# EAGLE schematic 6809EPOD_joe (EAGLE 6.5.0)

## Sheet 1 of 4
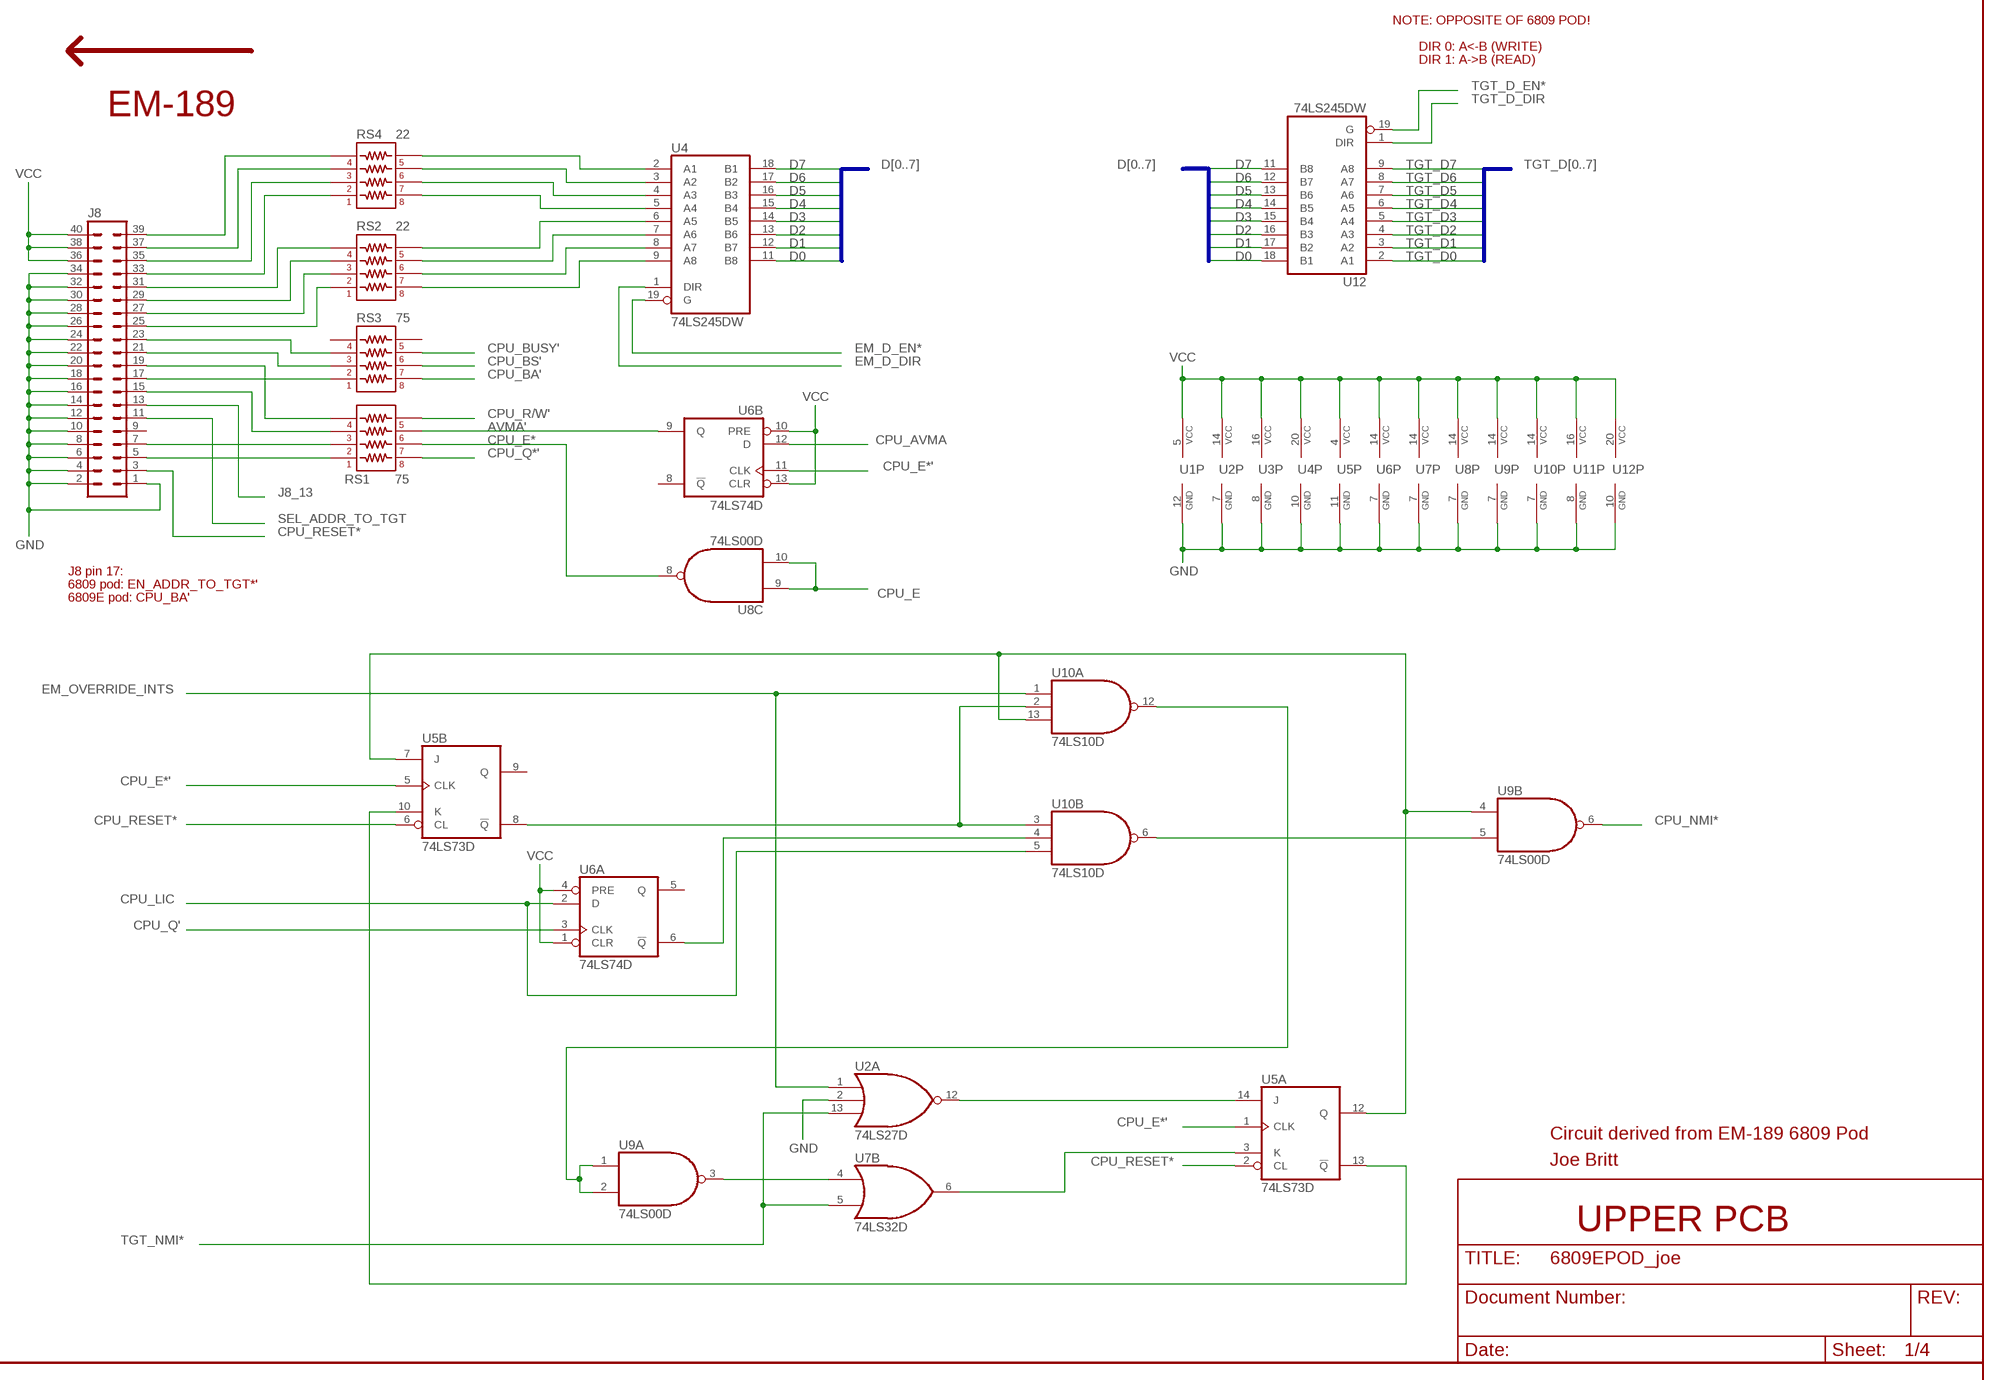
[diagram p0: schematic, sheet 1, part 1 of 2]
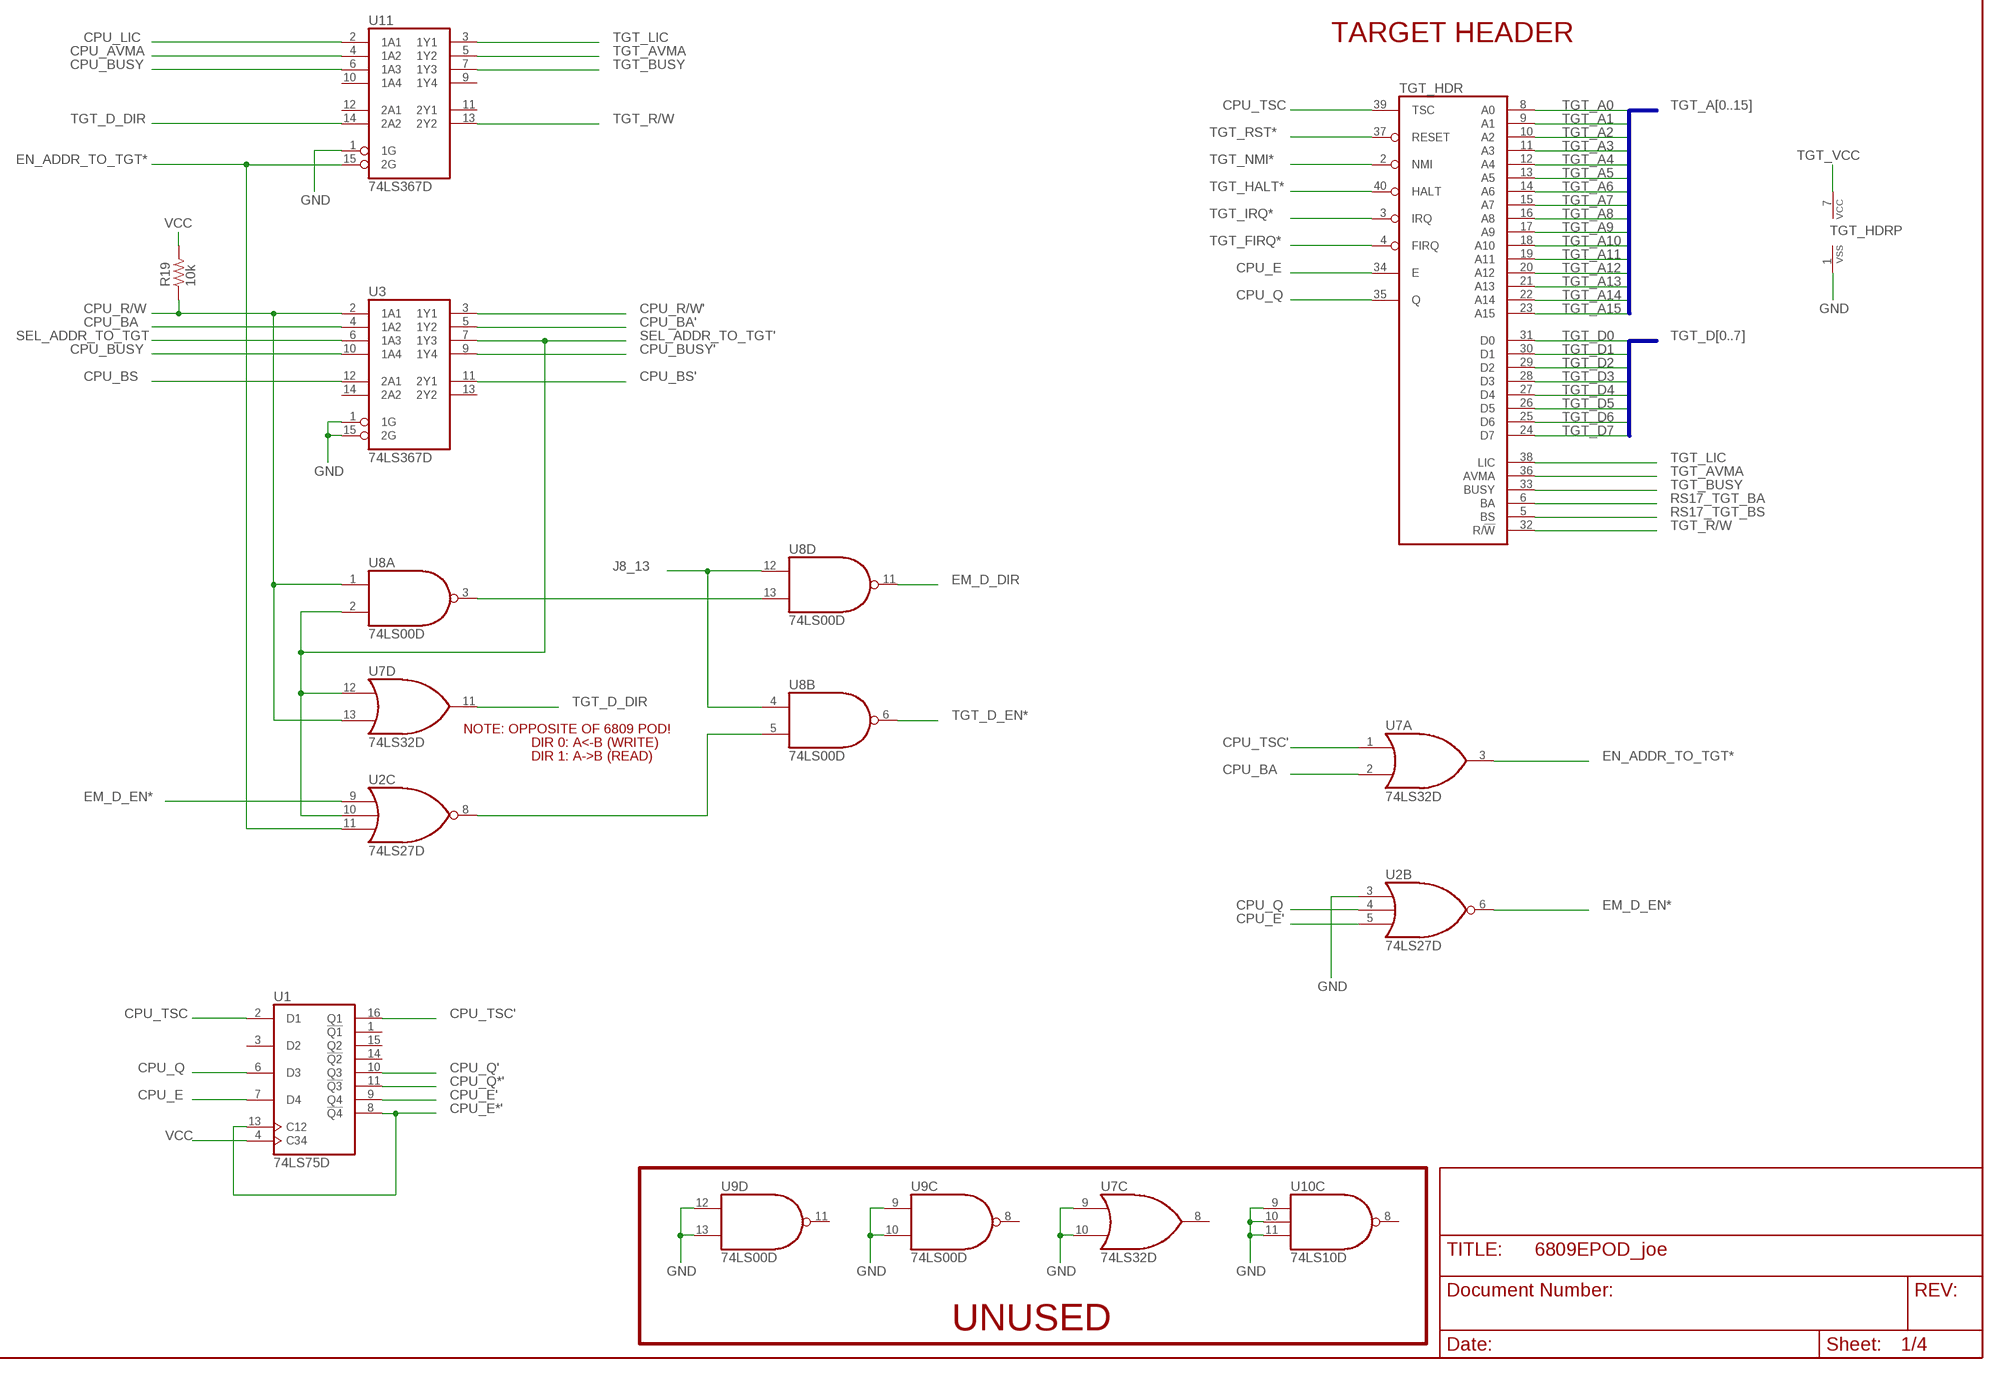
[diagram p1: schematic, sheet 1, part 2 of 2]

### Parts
J8  MA20-2  [MA20-2]
R19  10k  R_0603  [R0603]
RS1  75  V8V  [V8V]
RS2  22  V8V  [V8V]
RS3  75  V8V  [V8V]
RS4  22  V8V  [V8V]
TGT_HDR  6809EHDR40  [HDR40]
U1  74LS75D  [SO16]
U2  74LS27D  [SO14]
U3  74LS367D  [SO16]
U4  74LS245DW  [SO20W]
U5  74LS73D  [SO14]
U6  74LS74D  [SO14]
U7  74LS32D  [SO14]
U8  74LS00D  [SO14]
U9  74LS00D  [SO14]
U10  74LS10D  [SO14]
U11  74LS367D  [SO16]
U12  74LS245DW  [SO20W]

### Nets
AVMA': RS1.R3B U6.9(B:Q)
CPU_AVMA: U6.12(B:D) U11.4(1A2) ; also sheet 2
CPU_BA: U3.4(1A2) U7.2(A:I1) ; also sheet 2
CPU_BA': RS3.R1B U3.5(1Y2)
CPU_BS: U3.12(2A1) ; also sheet 2
CPU_BS': RS3.R2B U3.11(2Y1)
CPU_BUSY: U3.10(1A4) U11.6(1A3) ; also sheet 2
CPU_BUSY': RS3.R3B U3.9(1Y4)
CPU_E: TGT_HDR.34(E) U1.7(D4) U8.9(C:I0) U8.10(C:I1) ; also sheet 2
CPU_E': U1.9(Q4) U2.5(B:I2)
CPU_E*: RS1.R2B U8.8(C:O)
CPU_E*': U1.8(!Q4) U1.13(C12) U5.1(A:CLK) U5.5(B:CLK) U6.11(B:CLK)
CPU_LIC: U6.2(A:D) U10.5(B:I2) U11.2(1A1) ; also sheet 2
CPU_NMI*: U9.6(B:O) ; also sheet 2
CPU_Q: TGT_HDR.35(Q) U1.6(D3) U2.4(B:I1) ; also sheet 2
CPU_Q': U1.10(Q3) U6.3(A:CLK)
CPU_Q*': RS1.R1B U1.11(!Q3)
CPU_R/W: R19.1 U3.2(1A1) U7.13(D:I1) U8.1(A:I0) ; also sheet 2
CPU_R/W': RS1.R4B U3.3(1Y1)
CPU_RESET*: J8.3 U5.2(A:CL) U5.6(B:CL) ; also sheet 2
CPU_TSC: TGT_HDR.39(TSC) U1.2(D1) ; also sheet 2
CPU_TSC': U1.16(Q1) U7.1(A:I0)
D0: U4.11(B8) U12.18(B1) ; also sheet 2
D1: U4.12(B7) U12.17(B2) ; also sheet 2
D2: U4.13(B6) U12.16(B3) ; also sheet 2
D3: U4.14(B5) U12.15(B4) ; also sheet 2
D4: U4.15(B4) U12.14(B5) ; also sheet 2
D5: U4.16(B3) U12.13(B6) ; also sheet 2
D6: U4.17(B2) U12.12(B7) ; also sheet 2
D7: U4.18(B1) U12.11(B8) ; also sheet 2
EM_D_DIR: U4.1(DIR) U8.11(D:O)
EM_D_EN*: U2.6(B:O) U2.9(C:I0) U4.19(G)
EM_OVERRIDE_INTS: U2.1(A:I0) U10.1(A:I0) ; also sheet 2
EN_ADDR_TO_TGT*: U2.11(C:I2) U7.3(A:O) U11.15(2G) ; also sheet 2
GND: J8.1 J8.2 J8.4 J8.6 J8.8 J8.10 J8.12 J8.14 J8.16 J8.18 J8.20 J8.22 J8.24 J8.26 J8.28 J8.30 J8.32 J8.34 TGT_HDR.1(VSS) U1.12(GND) U2.2(A:I1) U2.3(B:I0) U2.7(P:GND) U3.1(1G) U3.8(GND) U3.15(2G) U4.10(GND) U5.11(P:GND) U6.7(P:GND) U7.7(P:GND) U7.9(C:I0) U7.10(C:I1) U8.7(P:GND) U9.7(P:GND) U9.9(C:I0) U9.10(C:I1) U9.12(D:I0) U9.13(D:I1) U10.7(P:GND) U10.9(C:I0) U10.10(C:I1) U10.11(C:I2) U11.1(1G) U11.8(GND) U12.10(GND) ; also sheet 2,3
J8_13: J8.13 U8.4(B:I0) U8.12(D:I0)
N$2: J8.5 RS1.R1A
N$3: J8.7 RS1.R2A
N$4: J8.15 RS1.R3A
N$5: J8.19 RS1.R4A
N$6: J8.17 RS3.R1A
N$7: J8.21 RS3.R2A
N$8: J8.23 RS3.R3A
N$9: J8.25 RS2.R1A
N$10: J8.27 RS2.R2A
N$11: J8.29 RS2.R3A
N$12: J8.31 RS2.R4A
N$13: J8.33 RS4.R1A
N$14: J8.35 RS4.R2A
N$15: J8.37 RS4.R3A
N$16: J8.39 RS4.R4A
N$17: RS2.R1B U4.9(A8)
N$18: RS2.R2B U4.8(A7)
N$19: RS2.R3B U4.7(A6)
N$20: RS2.R4B U4.6(A5)
N$21: RS4.R1B U4.5(A4)
N$22: RS4.R2B U4.4(A3)
N$23: RS4.R3B U4.3(A2)
N$24: RS4.R4B U4.2(A1)
N$45: U8.3(A:O) U8.13(D:I1)
N$46: U2.8(C:O) U8.5(B:I1)
N$124: U2.12(A:O) U5.14(A:J)
N$125: U5.8(B:!Q) U10.2(A:I1) U10.3(B:I0)
N$126: U6.6(A:!Q) U10.4(B:I1)
N$127: U5.10(B:K) U5.13(A:!Q)
N$128: U9.5(B:I1) U10.6(B:O)
N$129: U5.7(B:J) U5.12(A:Q) U9.4(B:I0) U10.13(A:I2)
N$130: U9.1(A:I0) U9.2(A:I1) U10.12(A:O)
N$131: U7.4(B:I0) U9.3(A:O)
N$132: U5.3(A:K) U7.6(B:O)
RS17_TGT_BA: TGT_HDR.6(BA) ; also sheet 2
RS17_TGT_BS: TGT_HDR.5(BS) ; also sheet 2
SEL_ADDR_TO_TGT: J8.11 U3.6(1A3)
SEL_ADDR_TO_TGT': U2.10(C:I1) U3.7(1Y3) U7.12(D:I0) U8.2(A:I1) ; also sheet 2
TGT_A0: TGT_HDR.8(A0) ; also sheet 2
TGT_A1: TGT_HDR.9(A1) ; also sheet 2
TGT_A2: TGT_HDR.10(A2) ; also sheet 2
TGT_A3: TGT_HDR.11(A3) ; also sheet 2
TGT_A4: TGT_HDR.12(A4) ; also sheet 2
TGT_A5: TGT_HDR.13(A5) ; also sheet 2
TGT_A6: TGT_HDR.14(A6) ; also sheet 2
TGT_A7: TGT_HDR.15(A7) ; also sheet 2
TGT_A8: TGT_HDR.16(A8) ; also sheet 2
TGT_A9: TGT_HDR.17(A9) ; also sheet 2
TGT_A10: TGT_HDR.18(A10) ; also sheet 2
TGT_A11: TGT_HDR.19(A11) ; also sheet 2
TGT_A12: TGT_HDR.20(A12) ; also sheet 2
TGT_A13: TGT_HDR.21(A13) ; also sheet 2
TGT_A14: TGT_HDR.22(A14) ; also sheet 2
TGT_A15: TGT_HDR.23(A15) ; also sheet 2
TGT_AVMA: TGT_HDR.36(AVMA) U11.5(1Y2)
TGT_BUSY: TGT_HDR.33(BUSY) U11.7(1Y3)
TGT_D0: TGT_HDR.31(D0) U12.2(A1)
TGT_D1: TGT_HDR.30(D1) U12.3(A2)
TGT_D2: TGT_HDR.29(D2) U12.4(A3)
TGT_D3: TGT_HDR.28(D3) U12.5(A4)
TGT_D4: TGT_HDR.27(D4) U12.6(A5)
TGT_D5: TGT_HDR.26(D5) U12.7(A6)
TGT_D6: TGT_HDR.25(D6) U12.8(A7)
TGT_D7: TGT_HDR.24(D7) U12.9(A8)
TGT_D_DIR: U7.11(D:O) U11.14(2A2) U12.1(DIR)
TGT_D_EN*: U8.6(B:O) U12.19(G)
TGT_FIRQ*: TGT_HDR.4(FIRQ) ; also sheet 2
TGT_HALT*: TGT_HDR.40(HALT) ; also sheet 2
TGT_IRQ*: TGT_HDR.3(IRQ) ; also sheet 2
TGT_LIC: TGT_HDR.38(LIC) U11.3(1Y1)
TGT_NMI*: TGT_HDR.2(NMI) U2.13(A:I2) U7.5(B:I1) ; also sheet 2
TGT_R/W: TGT_HDR.32(R/!W) U11.13(2Y2)
TGT_RST*: TGT_HDR.37(RESET) ; also sheet 2
TGT_VCC: TGT_HDR.7(VCC) ; also sheet 2,3
VCC: J8.36 J8.38 J8.40 R19.2 U1.4(C34) U1.5(VCC) U2.14(P:VCC) U3.16(VCC) U4.20(VCC) U5.4(P:VCC) U6.1(A:CLR) U6.4(A:PRE) U6.10(B:PRE) U6.13(B:CLR) U6.14(P:VCC) U7.14(P:VCC) U8.14(P:VCC) U9.14(P:VCC) U10.14(P:VCC) U11.16(VCC) U12.20(VCC) ; also sheet 2,3
Unconnected: J8.9 RS3.R4A RS3.R4B U1.1(!Q1) U1.3(D2) U1.14(!Q2) U1.15(Q2) U3.13(2Y2) U3.14(2A2) U5.9(B:Q) U6.5(A:Q) U6.8(B:!Q) U7.8(C:O) U9.8(C:O) U9.11(D:O) U10.8(C:O) U11.9(1Y4) U11.10(1A4) U11.11(2Y1) U11.12(2A1)

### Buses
D[0..7]
TGT_D[0..7]
TGT_A[0..15]

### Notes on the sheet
- NOTE: OPPOSITE OF 6809 POD!
- DIR 0: A<-B (WRITE)
- DIR 1: A->B (READ)
- EM-189
- J8 pin 17:
- 6809 pod: EN_ADDR_TO_TGT*'
- 6809E pod: CPU_BA'
- Circuit derived from EM-189 6809 Pod
- Joe Britt
- UPPER PCB
- TARGET HEADER
- NOTE: OPPOSITE OF 6809 POD!
- DIR 0: A<-B (WRITE)
- DIR 1: A->B (READ)
- UNUSED

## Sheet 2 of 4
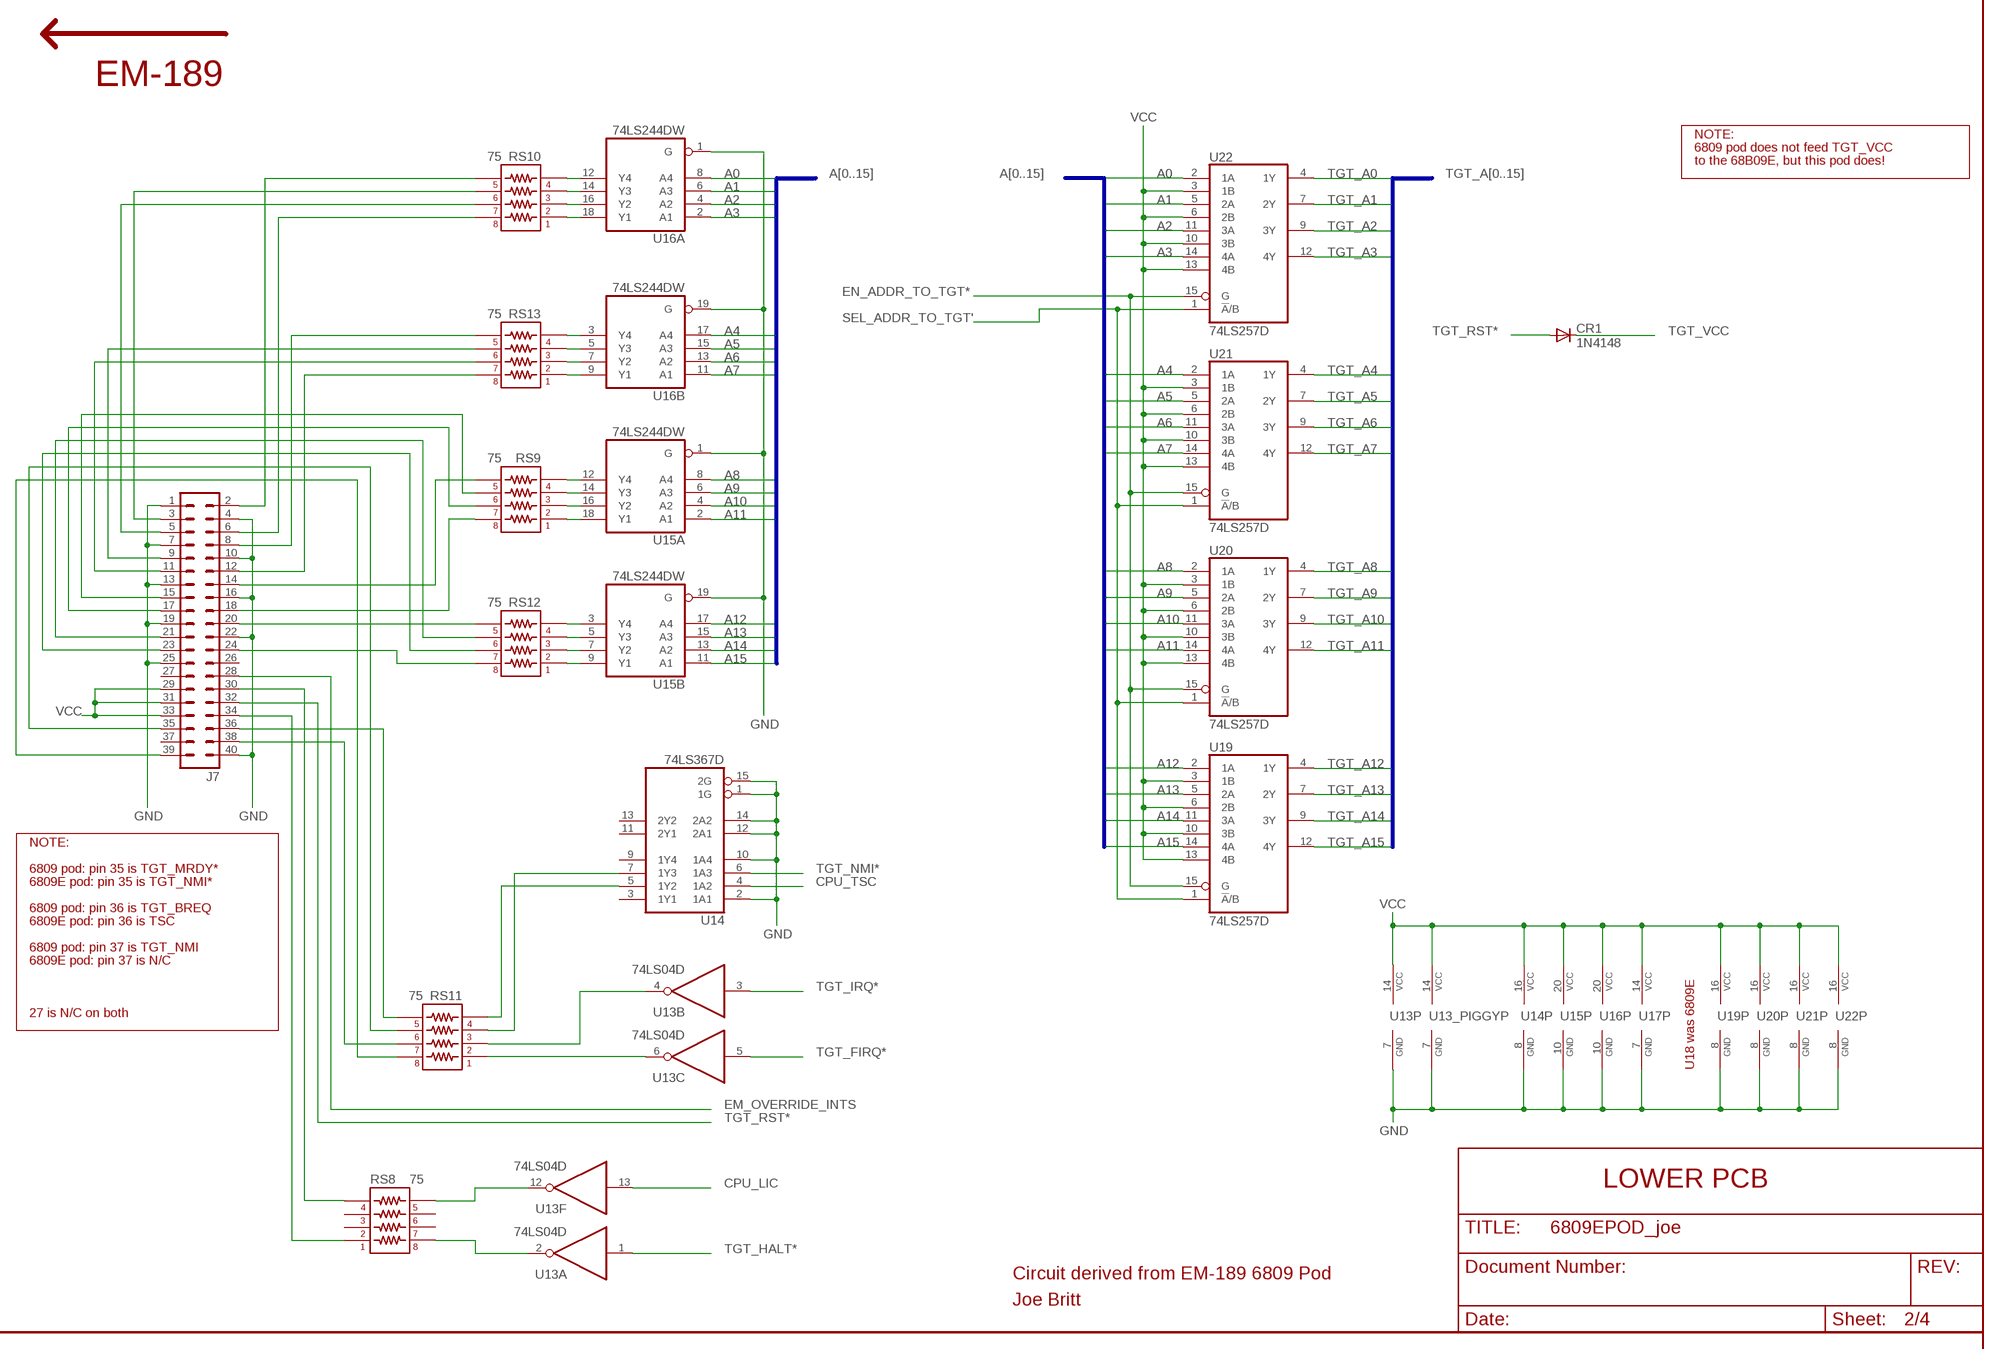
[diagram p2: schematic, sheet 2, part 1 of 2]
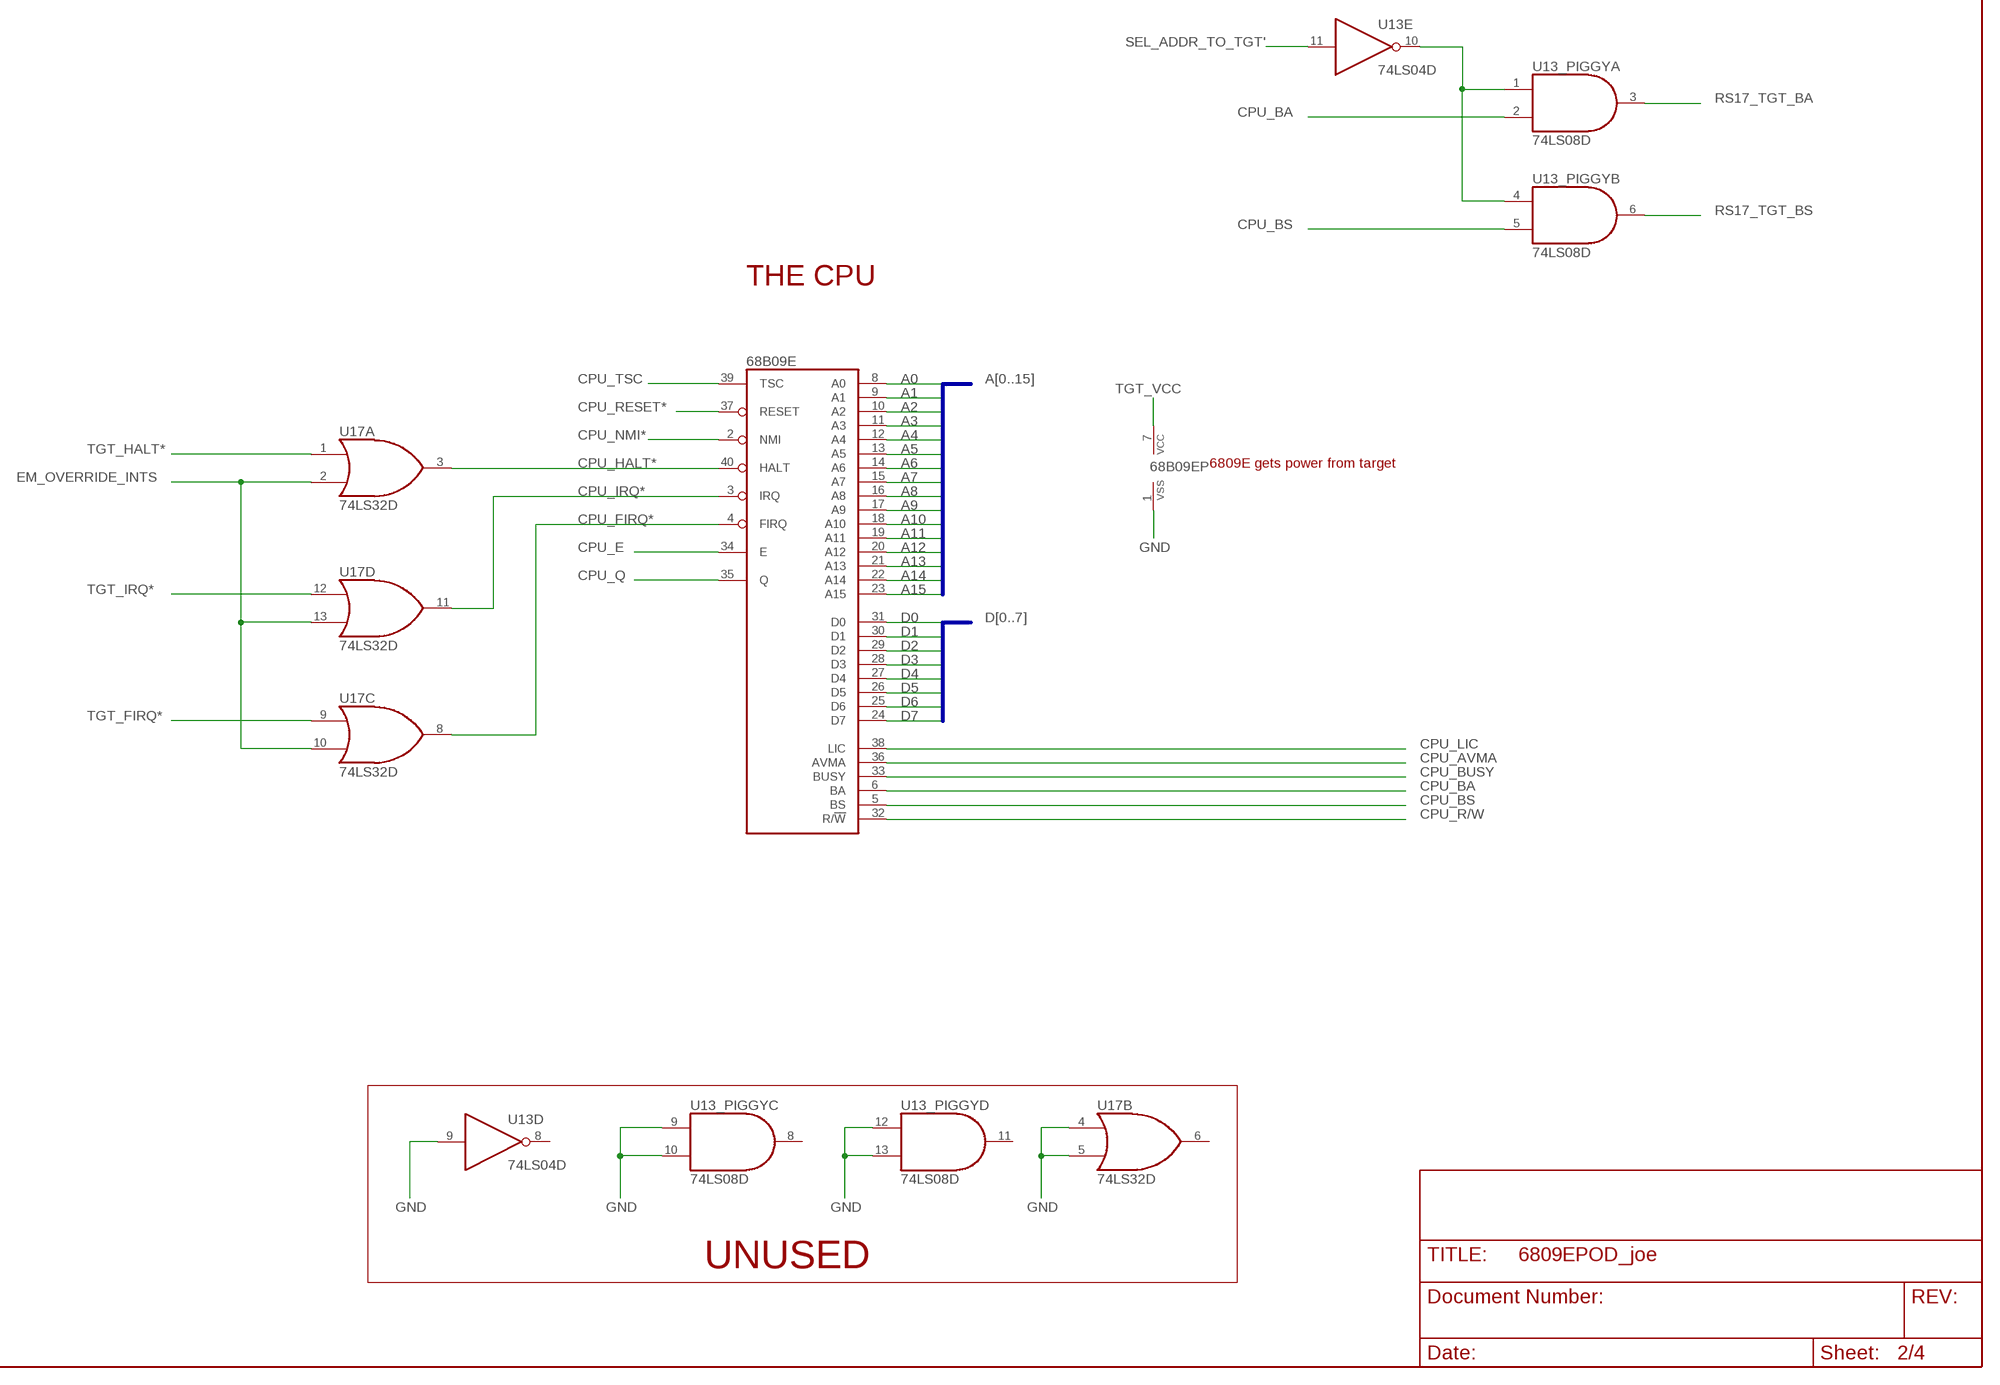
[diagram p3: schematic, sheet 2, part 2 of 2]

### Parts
68B09E  6809EDIP40  [DIL40]
CR1  1N4148  [DO35-10]
J7  MA20-2  [MA20-2]
RS8  75  V8V  [V8V]
RS9  75  V8V  [V8V]
RS10  75  V8V  [V8V]
RS11  75  V8V  [V8V]
RS12  75  V8V  [V8V]
RS13  75  V8V  [V8V]
U13  74LS04D  [SO14]
U13_PIGGY  74LS08D  [SO14]
U14  74LS367D  [SO16]
U15  74LS244DW  [SO20W]
U16  74LS244DW  [SO20W]
U17  74LS32D  [SO14]
U19  74LS257D  [SO16]
U20  74LS257D  [SO16]
U21  74LS257D  [SO16]
U22  74LS257D  [SO16]

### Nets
A0: 68B09E.8(A0) U16.8(A:A4) U22.2(1A)
A1: 68B09E.9(A1) U16.6(A:A3) U22.5(2A)
A2: 68B09E.10(A2) U16.4(A:A2) U22.11(3A)
A3: 68B09E.11(A3) U16.2(A:A1) U22.14(4A)
A4: 68B09E.12(A4) U16.17(B:A4) U21.2(1A)
A5: 68B09E.13(A5) U16.15(B:A3) U21.5(2A)
A6: 68B09E.14(A6) U16.13(B:A2) U21.11(3A)
A7: 68B09E.15(A7) U16.11(B:A1) U21.14(4A)
A8: 68B09E.16(A8) U15.8(A:A4) U20.2(1A)
A9: 68B09E.17(A9) U15.6(A:A3) U20.5(2A)
A10: 68B09E.18(A10) U15.4(A:A2) U20.11(3A)
A11: 68B09E.19(A11) U15.2(A:A1) U20.14(4A)
A12: 68B09E.20(A12) U15.17(B:A4) U19.2(1A)
A13: 68B09E.21(A13) U15.15(B:A3) U19.5(2A)
A14: 68B09E.22(A14) U15.13(B:A2) U19.11(3A)
A15: 68B09E.23(A15) U15.11(B:A1) U19.14(4A)
CPU_AVMA: 68B09E.36(AVMA) ; also sheet 1
CPU_BA: 68B09E.6(BA) U13_PIGGY.2(A:I1) ; also sheet 1
CPU_BS: 68B09E.5(BS) U13_PIGGY.5(B:I1) ; also sheet 1
CPU_BUSY: 68B09E.33(BUSY) ; also sheet 1
CPU_E: 68B09E.34(E) ; also sheet 1
CPU_FIRQ*: 68B09E.4(FIRQ) U17.8(C:O)
CPU_HALT*: 68B09E.40(HALT) U17.3(A:O)
CPU_IRQ*: 68B09E.3(IRQ) U17.11(D:O)
CPU_LIC: 68B09E.38(LIC) U13.13(F:I) ; also sheet 1
CPU_NMI*: 68B09E.2(NMI) ; also sheet 1
CPU_Q: 68B09E.35(Q) ; also sheet 1
CPU_R/W: 68B09E.32(R/!W) ; also sheet 1
CPU_RESET*: 68B09E.37(RESET) ; also sheet 1
CPU_TSC: 68B09E.39(TSC) U14.4(1A2) ; also sheet 1
D0: 68B09E.31(D0) ; also sheet 1
D1: 68B09E.30(D1) ; also sheet 1
D2: 68B09E.29(D2) ; also sheet 1
D3: 68B09E.28(D3) ; also sheet 1
D4: 68B09E.27(D4) ; also sheet 1
D5: 68B09E.26(D5) ; also sheet 1
D6: 68B09E.25(D6) ; also sheet 1
D7: 68B09E.24(D7) ; also sheet 1
EM_OVERRIDE_INTS: J7.28 U17.2(A:I1) U17.10(C:I1) U17.13(D:I1) ; also sheet 1
EN_ADDR_TO_TGT*: U19.15(G) U20.15(G) U21.15(G) U22.15(G) ; also sheet 1
GND: 68B09E.1(VSS) J7.1 J7.4 J7.7 J7.10 J7.13 J7.16 J7.19 J7.22 J7.25 J7.40 U13.7(P:GND) U13.9(D:I) U13_PIGGY.7(P:GND) U13_PIGGY.9(C:I0) U13_PIGGY.10(C:I1) U13_PIGGY.12(D:I0) U13_PIGGY.13(D:I1) U14.1(1G) U14.2(1A1) U14.8(GND) U14.10(1A4) U14.12(2A1) U14.14(2A2) U14.15(2G) U15.1(A:G) U15.10(P:GND) U15.19(B:G) U16.1(A:G) U16.10(P:GND) U16.19(B:G) U17.4(B:I0) U17.5(B:I1) U17.7(P:GND) U19.8(GND) U20.8(GND) U21.8(GND) U22.8(GND) ; also sheet 1,3
N$61: J7.3 RS10.R3B
N$62: J7.5 RS10.R2B
N$81: J7.9 RS13.R3B
N$82: J7.11 RS13.R2B
N$83: J7.15 RS9.R3B
N$84: J7.17 RS9.R2B
N$85: J7.21 RS12.R3B
N$86: J7.23 RS12.R2B
N$87: J7.35 RS11.R3B
N$88: J7.39 RS11.R1B
N$89: J7.2 RS10.R4B
N$90: J7.6 RS10.R1B
N$91: J7.8 RS13.R4B
N$92: J7.12 RS13.R1B
N$93: J7.18 RS9.R1B
N$94: J7.14 RS9.R4B
N$95: J7.20 RS12.R4B
N$96: J7.24 RS12.R1B
N$97: J7.30 RS8.R4A
N$98: J7.34 RS8.R1A
N$99: J7.36 RS11.R4B
N$100: J7.38 RS11.R2B
N$101: RS10.R4A U16.12(A:Y4)
N$102: RS10.R3A U16.14(A:Y3)
N$103: RS10.R2A U16.16(A:Y2)
N$104: RS10.R1A U16.18(A:Y1)
N$105: RS13.R4A U16.3(B:Y4)
N$106: RS13.R3A U16.5(B:Y3)
N$107: RS13.R2A U16.7(B:Y2)
N$108: RS13.R1A U16.9(B:Y1)
N$109: RS9.R4A U15.12(A:Y4)
N$110: RS9.R3A U15.14(A:Y3)
N$111: RS9.R2A U15.16(A:Y2)
N$112: RS9.R1A U15.18(A:Y1)
N$113: RS12.R4A U15.3(B:Y4)
N$114: RS12.R3A U15.5(B:Y3)
N$115: RS12.R2A U15.7(B:Y2)
N$116: RS12.R1A U15.9(B:Y1)
N$117: U13.10(E:O) U13_PIGGY.1(A:I0) U13_PIGGY.4(B:I0)
N$118: RS8.R1B U13.2(A:O)
N$119: RS11.R2A U13.4(B:O)
N$120: RS11.R1A U13.6(C:O)
N$121: RS8.R4B U13.12(F:O)
N$122: RS11.R4A U14.5(1Y2)
N$123: RS11.R3A U14.7(1Y3)
RS17_TGT_BA: U13_PIGGY.3(A:O) ; also sheet 1
RS17_TGT_BS: U13_PIGGY.6(B:O) ; also sheet 1
SEL_ADDR_TO_TGT': U13.11(E:I) U19.1(!A!/B) U20.1(!A!/B) U21.1(!A!/B) U22.1(!A!/B) ; also sheet 1
TGT_A0: U22.4(1Y) ; also sheet 1
TGT_A1: U22.7(2Y) ; also sheet 1
TGT_A2: U22.9(3Y) ; also sheet 1
TGT_A3: U22.12(4Y) ; also sheet 1
TGT_A4: U21.4(1Y) ; also sheet 1
TGT_A5: U21.7(2Y) ; also sheet 1
TGT_A6: U21.9(3Y) ; also sheet 1
TGT_A7: U21.12(4Y) ; also sheet 1
TGT_A8: U20.4(1Y) ; also sheet 1
TGT_A9: U20.7(2Y) ; also sheet 1
TGT_A10: U20.9(3Y) ; also sheet 1
TGT_A11: U20.12(4Y) ; also sheet 1
TGT_A12: U19.4(1Y) ; also sheet 1
TGT_A13: U19.7(2Y) ; also sheet 1
TGT_A14: U19.9(3Y) ; also sheet 1
TGT_A15: U19.12(4Y) ; also sheet 1
TGT_FIRQ*: U13.5(C:I) U17.9(C:I0) ; also sheet 1
TGT_HALT*: U13.1(A:I) U17.1(A:I0) ; also sheet 1
TGT_IRQ*: U13.3(B:I) U17.12(D:I0) ; also sheet 1
TGT_NMI*: U14.6(1A3) ; also sheet 1
TGT_RST*: CR1.A J7.32 ; also sheet 1
TGT_VCC: 68B09E.7(VCC) CR1.C ; also sheet 1,3
VCC: J7.29 J7.31 J7.33 U13.14(P:VCC) U13_PIGGY.14(P:VCC) U14.16(VCC) U15.20(P:VCC) U16.20(P:VCC) U17.14(P:VCC) U19.3(1B) U19.6(2B) U19.10(3B) U19.13(4B) U19.16(VCC) U20.3(1B) U20.6(2B) U20.10(3B) U20.13(4B) U20.16(VCC) U21.3(1B) U21.6(2B) U21.10(3B) U21.13(4B) U21.16(VCC) U22.3(1B) U22.6(2B) U22.10(3B) U22.13(4B) U22.16(VCC) ; also sheet 1,3
Unconnected: J7.26 J7.27 J7.37 RS8.R2A RS8.R2B RS8.R3A RS8.R3B U13.8(D:O) U13_PIGGY.8(C:O) U13_PIGGY.11(D:O) U14.3(1Y1) U14.9(1Y4) U14.11(2Y1) U14.13(2Y2) U17.6(B:O)

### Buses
A[0..15]
D[0..7]
TGT_A[0..15]

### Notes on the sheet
- EM-189
- NOTE:
- 6809 pod does not feed TGT_VCC
- to the 68B09E, but this pod does!
- NOTE:
- 6809 pod: pin 35 is TGT_MRDY*
- 6809E pod: pin 35 is TGT_NMI*
- 6809 pod: pin 36 is TGT_BREQ
- 6809E pod: pin 36 is TSC
- 6809 pod: pin 37 is TGT_NMI
- 6809E pod: pin 37 is N/C
- 27 is N/C on both
- U18 was 6809E
- LOWER PCB
- Circuit derived from EM-189 6809 Pod
- Joe Britt
- THE CPU
- 6809E gets power from target
- UNUSED

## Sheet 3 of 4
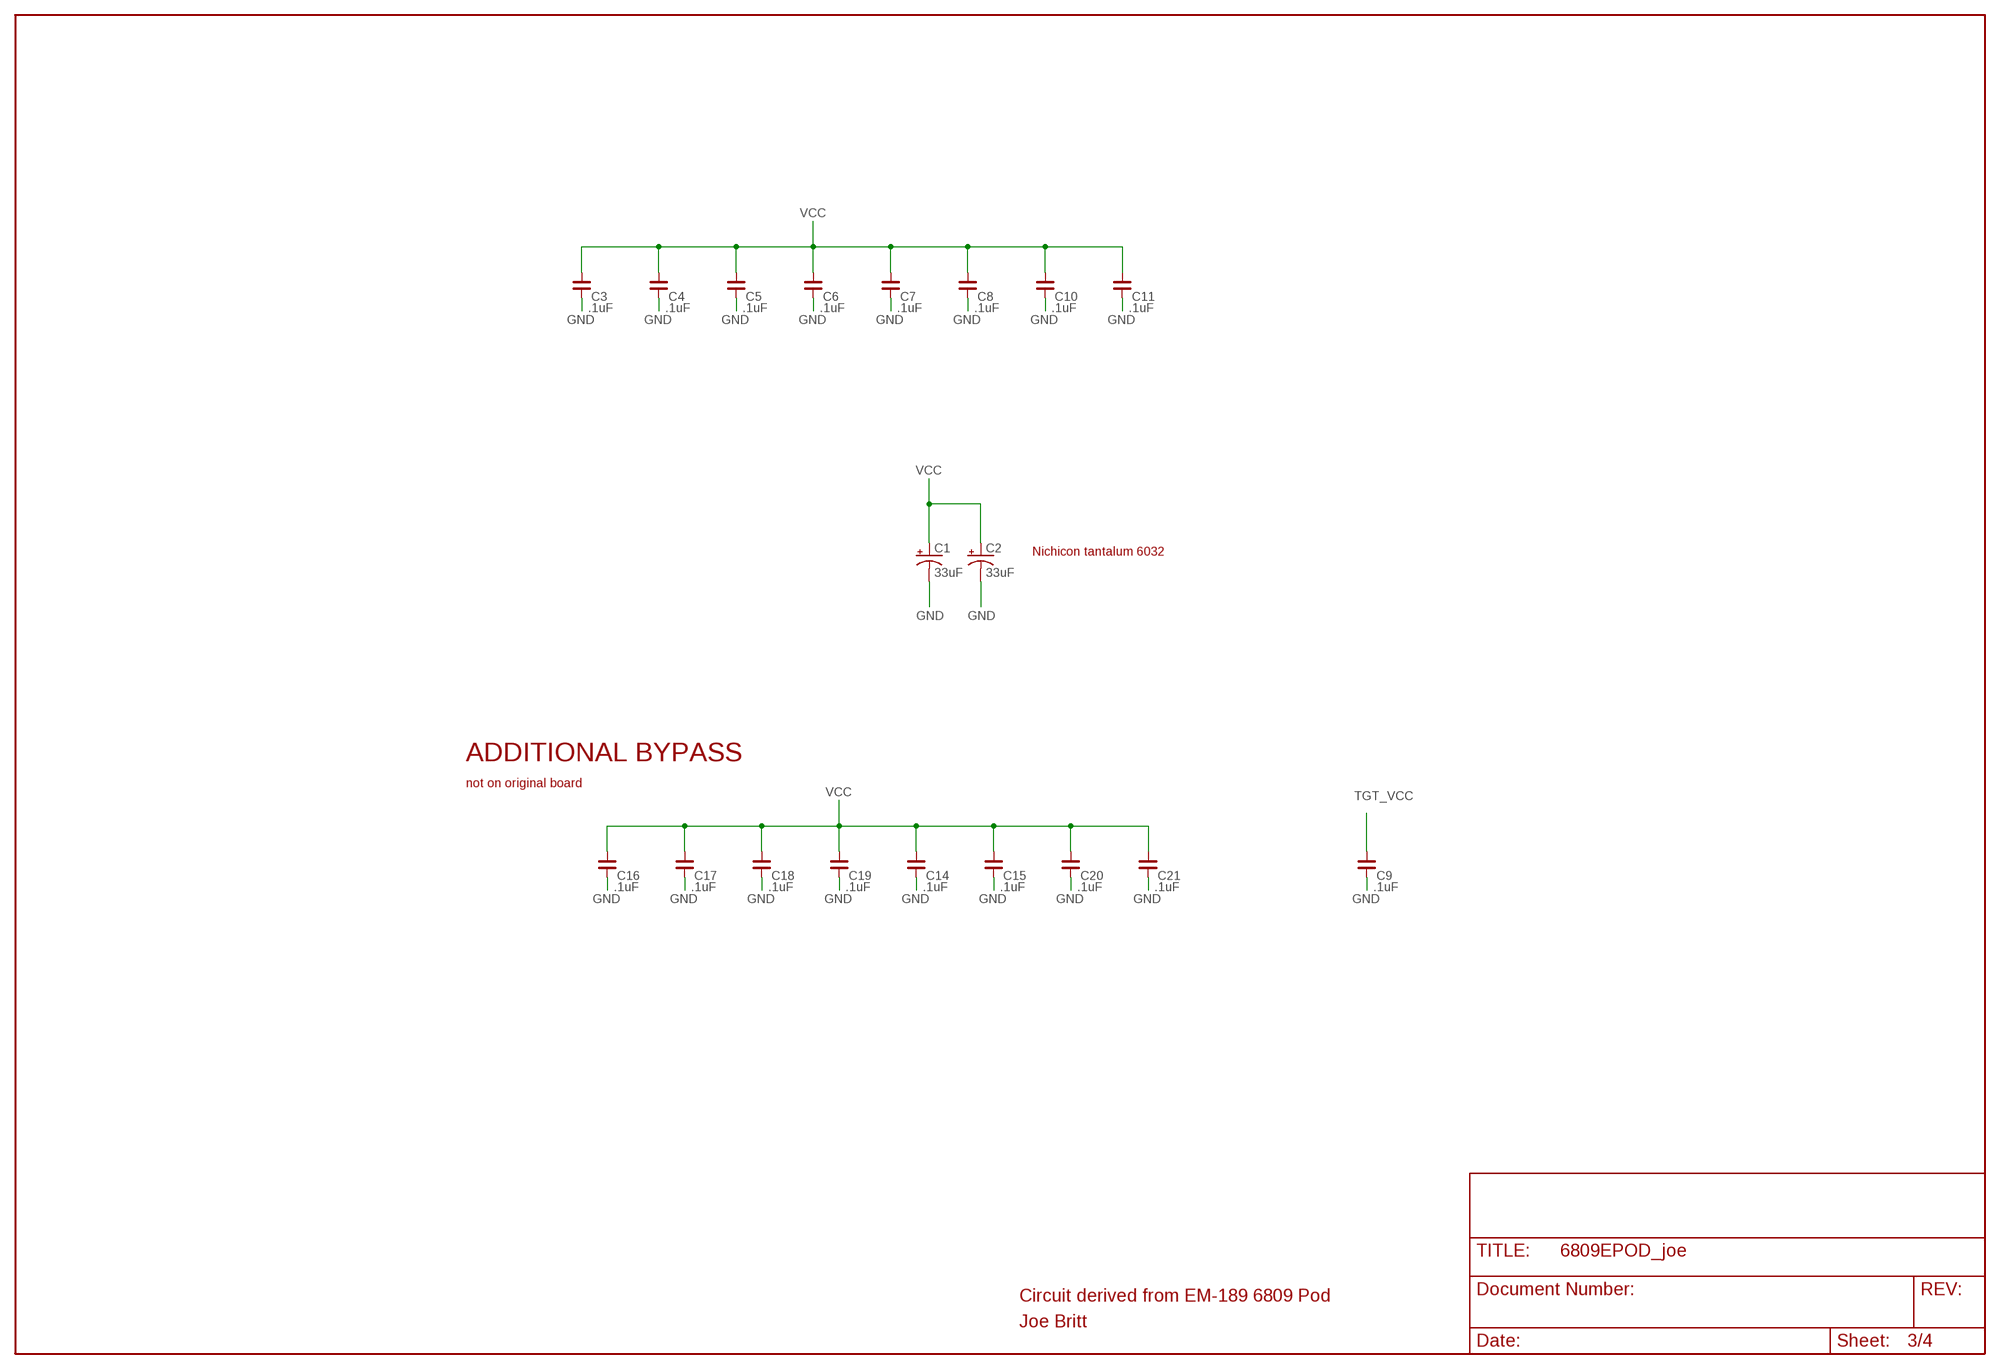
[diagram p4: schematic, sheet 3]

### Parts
C1  33uF  CPOL-USCT6032  [CT6032]
C2  33uF  CPOL-USCT6032  [CT6032]
C3  .1uF  C_0603  [C0603]
C4  .1uF  C_0603  [C0603]
C5  .1uF  C_0603  [C0603]
C6  .1uF  C_0603  [C0603]
C7  .1uF  C_0603  [C0603]
C8  .1uF  C_0603  [C0603]
C9  .1uF  C_0603  [C0603]
C10  .1uF  C_0603  [C0603]
C11  .1uF  C_0603  [C0603]
C14  .1uF  C_0603  [C0603]
C15  .1uF  C_0603  [C0603]
C16  .1uF  C_0603  [C0603]
C17  .1uF  C_0603  [C0603]
C18  .1uF  C_0603  [C0603]
C19  .1uF  C_0603  [C0603]
C20  .1uF  C_0603  [C0603]
C21  .1uF  C_0603  [C0603]

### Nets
GND: C1.- C2.- C3.2 C4.2 C5.2 C6.2 C7.2 C8.2 C9.2 C10.2 C11.2 C14.2 C15.2 C16.2 C17.2 C18.2 C19.2 C20.2 C21.2 ; also sheet 1,2
TGT_VCC: C9.1 ; also sheet 1,2
VCC: C1.+ C2.+ C3.1 C4.1 C5.1 C6.1 C7.1 C8.1 C10.1 C11.1 C14.1 C15.1 C16.1 C17.1 C18.1 C19.1 C20.1 C21.1 ; also sheet 1,2

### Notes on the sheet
- Nichicon tantalum 6032
- ADDITIONAL BYPASS
- not on original board
- Circuit derived from EM-189 6809 Pod
- Joe Britt

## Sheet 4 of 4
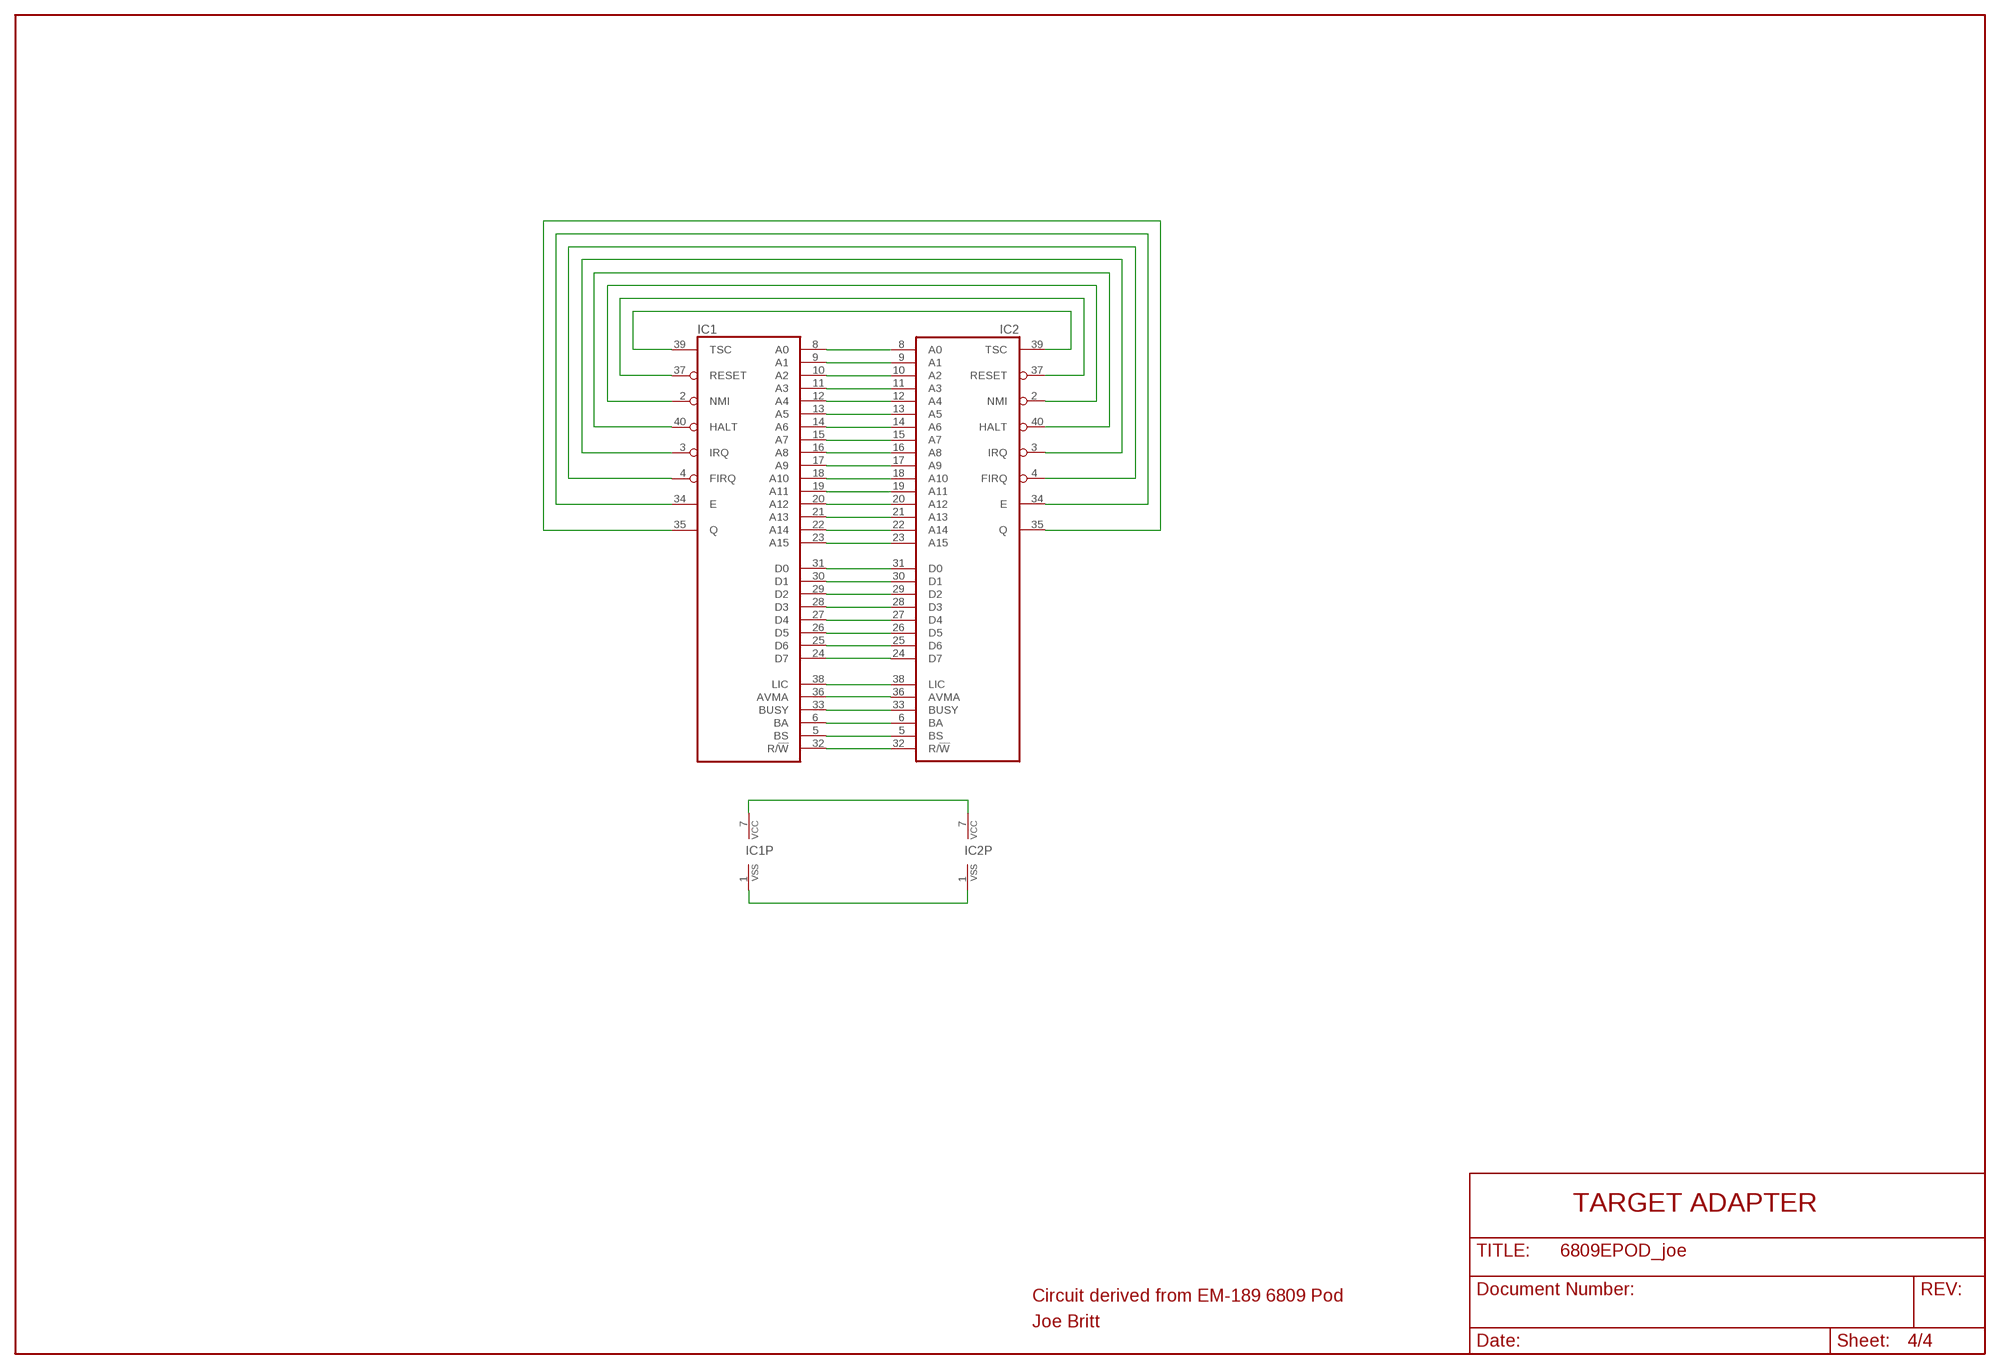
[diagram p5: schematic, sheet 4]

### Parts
IC1  6809EDIP40  [DIL40]
IC2  6809EHDR40  [HDR40]

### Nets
N$25: IC1.8(A0) IC2.8(A0)
N$26: IC1.9(A1) IC2.9(A1)
N$27: IC1.10(A2) IC2.10(A2)
N$28: IC1.11(A3) IC2.11(A3)
N$29: IC1.12(A4) IC2.12(A4)
N$30: IC1.13(A5) IC2.13(A5)
N$31: IC1.14(A6) IC2.14(A6)
N$32: IC1.15(A7) IC2.15(A7)
N$33: IC1.16(A8) IC2.16(A8)
N$34: IC1.17(A9) IC2.17(A9)
N$35: IC1.18(A10) IC2.18(A10)
N$36: IC1.19(A11) IC2.19(A11)
N$37: IC1.20(A12) IC2.20(A12)
N$38: IC1.21(A13) IC2.21(A13)
N$39: IC1.22(A14) IC2.22(A14)
N$40: IC1.23(A15) IC2.23(A15)
N$41: IC1.31(D0) IC2.31(D0)
N$42: IC1.30(D1) IC2.30(D1)
N$43: IC1.29(D2) IC2.29(D2)
N$44: IC1.28(D3) IC2.28(D3)
N$47: IC1.27(D4) IC2.27(D4)
N$48: IC1.26(D5) IC2.26(D5)
N$49: IC1.25(D6) IC2.25(D6)
N$50: IC1.24(D7) IC2.24(D7)
N$51: IC1.38(LIC) IC2.38(LIC)
N$52: IC1.36(AVMA) IC2.36(AVMA)
N$53: IC1.33(BUSY) IC2.33(BUSY)
N$54: IC1.6(BA) IC2.6(BA)
N$55: IC1.5(BS) IC2.5(BS)
N$56: IC1.32(R/!W) IC2.32(R/!W)
N$57: IC1.39(TSC) IC2.39(TSC)
N$58: IC1.37(RESET) IC2.37(RESET)
N$59: IC1.2(NMI) IC2.2(NMI)
N$60: IC1.40(HALT) IC2.40(HALT)
N$63: IC1.3(IRQ) IC2.3(IRQ)
N$64: IC1.4(FIRQ) IC2.4(FIRQ)
N$65: IC1.34(E) IC2.34(E)
N$66: IC1.35(Q) IC2.35(Q)
N$67: IC1.7(VCC) IC2.7(VCC)
N$68: IC1.1(VSS) IC2.1(VSS)

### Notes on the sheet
- TARGET ADAPTER
- Circuit derived from EM-189 6809 Pod
- Joe Britt

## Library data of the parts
68B09E IC1 IC2 TGT_HDR = micro-motorola:6809E: MICROCONTROLLER/MEMORY DEVICE
C1 C2 = rcl:CPOL-US: POLARIZED CAPACITOR, American symbol
C3-C11 C14-C21 = rc-master-smd:C_: NON-POLARIZED CAP
CR1 = diode:1N4148: DIODE
J7 J8 = con-lstb:MA20-2: PIN HEADER
R19 = rc-master-smd:R_: RESISTOR
RS1-RS4 RS8-RS13 = pana_rpack:V8V
U1 = 74xx-us:74*75: 4-bit bistable LATCH
U2 = 74xx-us:74*27: Triple 3-input NOR gate
U3 U11 U14 = 74xx-us:74*367: Hex BUS DRIVER, 3-state
U4 U12 = 74xx-us:74*245: Octal BUS TRANSCEIVER, 3-state
U5 = 74xx-us:74*73: Dual J-K FLIP FLOP, clear
U6 = 74xx-us:74*74: Dual D type positive edge triggered FLIP FLOP, preset and clear
U7 U17 = 74xx-us:74*32: Quad 2-input OR gate
U8 U9 = 74xx-us:74*00: Quad 2-input NAND gate
U10 = 74xx-us:74*10: Triple 3-input NAND gate
U13 = 74xx-us:74*04: Hex INVERTER
U13_PIGGY = 74xx-us:74*08: Quad 2-input AND gate
U15 U16 = 74xx-us:74*244: Octal BUFFER and LINE DRIVER, 3-state
U19-U22 = 74xx-us:74*257: Quadruple 2-to 1 line data SELECTOR/MULTIPLEXER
